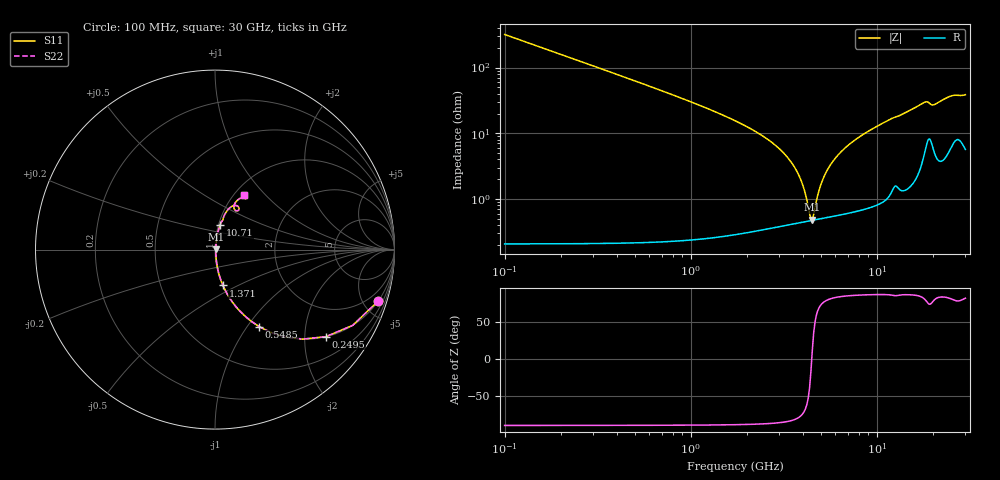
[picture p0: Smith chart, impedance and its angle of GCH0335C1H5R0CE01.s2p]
!Murata Part Number: GCH0335C1H5R0CE01
!These Parameters are Measured in Series Mode Connection
!Data Generated on Jun 19, 2026
!  o--ll--o
!Port1  Port2
!  o------o
!Operation Temp=25[degC], DC Bias Voltage=0[V]
!Freq. Start=100[MHz] Stop=30[GHz] 401[Steps]
# Hz S RI R 50
!Freq.(Hz) S11(Real) S11(Imag) S21(Real) S21(Imag) S12(Real) S12(Imag) S22(Real) S22(Imag)
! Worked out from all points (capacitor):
!   401 points, 100 MHz to 30 GHz, reference 50 ohm
!   read as one part in series: C = 5 pF near 249.5 MHz
!   lowest |Z| = 485 mohm at 4.51 GHz (marker M1)
!   series resonance near 4.48 GHz, so ESL is about 250 pH
!   S11 on the Smith chart (normalised r, x): 100 MHz: 1.00, -6.36; 249.5 MHz: 1.00, -2.54; 548.5 MHz: 1.00, -1.14; 1.371 GHz: 1.01, -0.42; 10.71 GHz: 1.02, +0.28; 30 GHz: 1.11, +0.76
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1e8  0.9099 -0.286  0.0901 0.286  0.0901 0.286  0.9099 -0.286
2.495e8  0.6177 -0.4851  0.3823 0.4851  0.3823 0.4851  0.6177 -0.4851
3.99e8  0.3853 -0.4853  0.6147 0.4853  0.6147 0.4853  0.3853 -0.4853
5.485e8  0.2469 -0.4293  0.7531 0.4293  0.7531 0.4293  0.2469 -0.4293
8.475e8  0.1172 -0.3185  0.8828 0.3185  0.8828 0.3185  0.1172 -0.3185
1.37075e9  0.0445 -0.2  0.9555 0.2  0.9555 0.2  0.0445 -0.2
2.86575e9  0.00787 -0.0643  0.9921 0.0643  0.9921 0.0643  0.00787 -0.0643
3.46375e9  0.00542 -0.0362  0.9946 0.0362  0.9946 0.0362  0.00542 -0.0362
3.91225e9  0.00474 -0.0189  0.9953 0.0189  0.9953 0.0189  0.00474 -0.0189
4.36075e9  0.00466 -0.00375  0.9953 0.00375  0.9953 0.00375  0.00466 -0.00375
4.51025e9  0.00473 0.000938  0.9953 -0.000938  0.9953 -0.000938  0.00473 0.000938
5.10825e9  0.00539 0.0183  0.9946 -0.0183  0.9946 -0.0183  0.00539 0.0183
5.781e9  0.00669 0.0357  0.9933 -0.0357  0.9933 -0.0357  0.00669 0.0357
6.75275e9  0.00933 0.0584  0.9907 -0.0584  0.9907 -0.0584  0.00933 0.0584
8.173e9  0.0145 0.088  0.9855 -0.088  0.9855 -0.088  0.0145 0.088
1.01165e10  0.0241 0.1249  0.9759 -0.1249  0.9759 -0.1249  0.0241 0.1249
1.07145e10  0.0277 0.1358  0.9723 -0.1358  0.9723 -0.1358  0.0277 0.1358
1.505e10  0.0598 0.2055  0.9402 -0.2055  0.9402 -0.2055  0.0598 0.2055
1.811475e10  0.1166 0.2457  0.8834 -0.2457  0.8834 -0.2457  0.1166 0.2457
2.005825e10  0.1113 0.2201  0.8887 -0.2201  0.8887 -0.2201  0.1113 0.2201
2.50665e10  0.1557 0.2899  0.8443 -0.2899  0.8443 -0.2899  0.1557 0.2899
3e10  0.1633 0.3026  0.8367 -0.3026  0.8367 -0.3026  0.1633 0.3026
